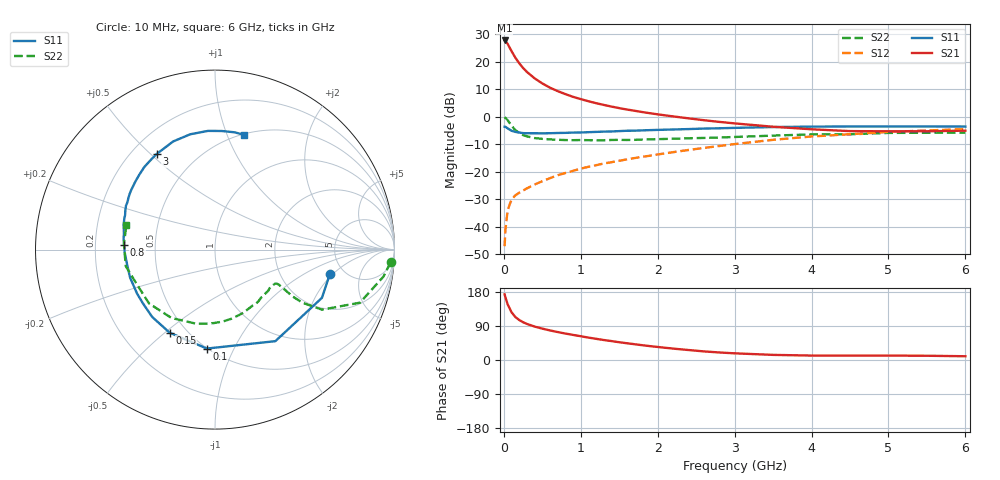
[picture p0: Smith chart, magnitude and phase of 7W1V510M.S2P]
! Infineon Technologies  Discrete & RF Semiconductors
! BFS17W
! Si NPN RF Bipolar Junction Transistor in SOT323
! VCE = 1.5 V  IC = 10 mA
! Common Emitter S-Parameters:  August  1999
# GHz  S  MA  R  50
!  f  S11  S21  S12  S22
! GHz  MAG  ANG  MAG  ANG  MAG  ANG  MAG  ANG
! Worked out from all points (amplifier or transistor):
!   36 points, 10 MHz to 6 GHz, reference 50 ohm
!   highest |S21| = 27.7 dB at 10 MHz (marker M1)
!   |S21| within 3 dB of that: start of sweep to 83.02 MHz
!   unconditionally stable (mu >= 1): 364 MHz to end of sweep
!   at 250 MHz: K = 0.84, MSG = 22.3 dB, |S12| = -26.9 dB
!   at 1.4 GHz: K = 1.27, MAG = 7.0 dB, |S12| = -16.6 dB
!   at 6 GHz: K = 1.10, MAG = -2.2 dB, |S12| = -4.5 dB
!   S11 on the Smith chart (normalised r, x): 10 MHz: 3.85, -1.85; 100 MHz: 0.50, -0.79; 150 MHz: 0.40, -0.52; 800 MHz: 0.33, +0.02; 3 GHz: 0.30, +0.52; 6 GHz: 0.51, +1.15
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0.01  0.6543 -12.1  24.28 173.2  0.0044 80.8  0.9807 -4.2
0.02  0.6536 -24.3  23.83 165.6  0.0086 79.2  0.9506 -9.1
0.05  0.611 -56.6  20.94 146.7  0.02 66.6  0.8601 -20.1
0.1  0.5532 -94.7  15.53 126.0  0.031 54.3  0.6839 -29.3
0.15  0.5274 -118.6  11.77 113.3  0.037 50.5  0.5688 -31.3
0.2  0.5131 -133.0  9.347 105.5  0.0412 50.8  0.504 -31.1
0.25  0.501 -143.3  7.676 99.7  0.0452 50.6  0.4618 -30.2
0.3  0.4985 -150.7  6.5 95.2  0.0496 52.7  0.4377 -29.6
0.4  0.4982 -161.6  4.969 88.2  0.0582 55.3  0.4069 -28.8
0.5  0.4964 -168.8  4.015 82.8  0.0668 58.0  0.3938 -28.8
0.6  0.4988 -174.2  3.36 78.0  0.076 59.6  0.3848 -29.6
0.8  0.5066 177.2  2.565 69.8  0.0943 61.5  0.3746 -33.4
0.9  0.5123 173.8  2.29 66.2  0.1033 62.3  0.3727 -35.5
1.1  0.5209 167.2  1.903 59.1  0.1222 63.0  0.3726 -40.8
1.3  0.5339 161.2  1.63 52.7  0.1405 63.1  0.3715 -46.9
1.6  0.5531 153.7  1.345 44.2  0.1665 63.1  0.3759 -56.2
2.2  0.5831 139.7  1.009 30.1  0.2255 62.6  0.3963 -76.9
3  0.6237 121.5  0.753 17.6  0.3166 58.3  0.4262 -104.9
3.5  0.6461 111.2  0.654 13.5  0.3781 53.5  0.4515 -122.5
4.5  0.6625 93.4  0.545 11.5  0.4785 41.1  0.4769 -156.4
5.5  0.6625 80.6  0.542 11.2  0.5598 29.4  0.5083 176.7
6  0.6598 75.9  0.555 9.9  0.5923 23.8  0.5119 164.7
